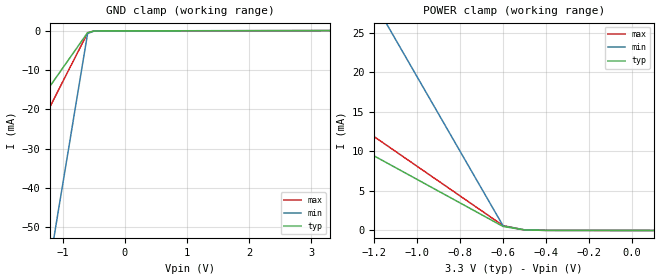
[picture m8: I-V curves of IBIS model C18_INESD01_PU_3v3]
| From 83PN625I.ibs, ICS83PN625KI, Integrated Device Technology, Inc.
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[Model] C18_INESD01_PU_3v3
Model_type   Input
Polarity   Non-Inverting
Vinl = 0.8V
Vinh = 2.0V
|   typ   min   max
C_comp   2pF   1.5pF   2.5pF
|   typ   min   max
[Voltage range]   3.3V   3.135V   3.465V
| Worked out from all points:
|   GND clamp passes 1 mA (typ) near -0.62 V on its own axis
|   POWER clamp passes 1 mA (typ) near -0.63 V on its own axis
[GND_clamp]
|Voltage   I (typ)   I (min)   I (max)
-3.3V     -61.39mA   -259.7mA   -84.47mA
-2.9V     -52.37mA   -221.3mA   -72.05mA
-2.8V     -50.12mA   -211.7mA   -68.94mA
-2.3V     -38.84mA   -163.8mA   -53.41mA
-2.2V     -36.59mA   -154.2mA   -50.3mA
-1.2V     -14.05mA   -58.3mA    -19.24mA
-1.1V     -11.79mA   -48.71mA   -16.13mA
-600mV    -519.3uA   -757.2uA   -601.3uA
-500mV    -121.7uA   -129.2uA   -121.2uA
-400mV    -77.06uA   -71.62uA   -83.32uA
3.3V      10.04pA    3.091uA    503nA
[Power_clamp]
|Voltage   I (typ)   I (min)   I (max)
-3.3V     40.67mA    127.8mA    51.25mA
-2.3V     25.79mA    80.7mA     32.5mA
-2.2V     24.3mA     75.98mA    30.62mA
-2V       21.33mA    66.56mA    26.87mA
-1.9V     19.84mA    61.84mA    24.99mA
-1.2V     9.428mA    28.85mA    11.86mA
-1.1V     7.94mA     24.14mA    9.988mA
-600mV    501.9uA    575.2uA    609.4uA
-500mV    65.34uA    72.75uA    60.6uA
100mV     -1.999uA   -1.87uA    -2.123uA
